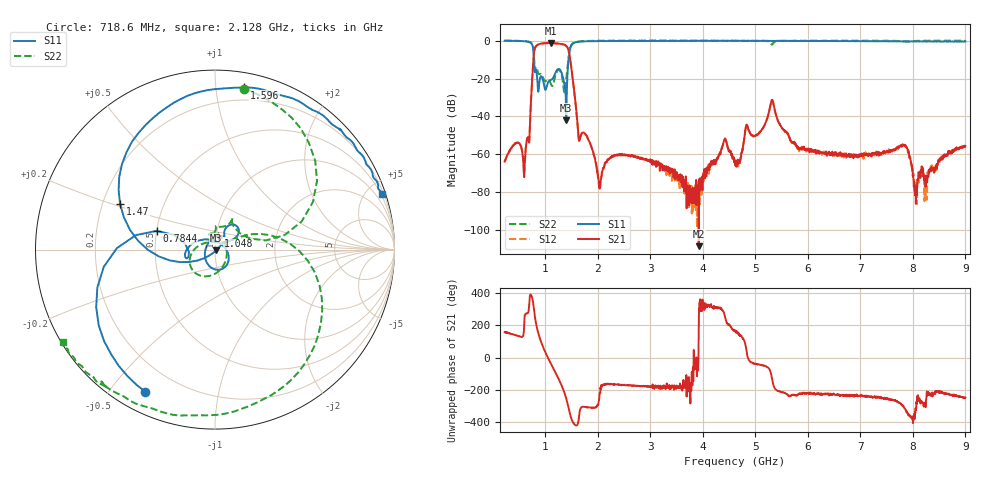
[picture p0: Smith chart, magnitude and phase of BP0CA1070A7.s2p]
!Agilent Technologies,E8358A,US41080443,A.07.50.56
!Agilent E8358A: A.07.50.56
!Date: Thursday, November 09, 2017 08:34:48
!Correction: S11(Full 2 Port(1,2))
!S21(Full 2 Port(1,2))
!S12(Full 2 Port(1,2))
!S22(Full 2 Port(1,2))
!S2P File: Measurements: S11, S21, S12, S22:
# Hz S  dB  R 50
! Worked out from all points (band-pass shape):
!   1601 points, 225 MHz to 9 GHz, reference 50 ohm
!   highest |S21| = -1.22 dB at 1.113 GHz (marker M1); lowest = -108.4 dB at 3.921 GHz (marker M2)
!   |S21| within 3 dB of the highest: 798.9 MHz to 1.432 GHz (632.8 MHz wide, 56.7 % of centre)
!   lowest |S11| = -42.0 dB at 1.399 GHz (marker M3), VSWR 1.02, Z = 50.7 - j0.309 ohm
!   |S11| at or under -10 dB: 785.7 MHz to 1.443 GHz (656.9 MHz wide, 59 % of centre)
!   |S22| runs from -27.3 to 0.1 dB; largest |S21 - S12| = 0.016
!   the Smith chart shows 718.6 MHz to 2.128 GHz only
!   S11 on the Smith chart (normalised r, x): 718.6 MHz: 0.09, -0.62; 784.4 MHz: 0.50, +0.12; 1.048 GHz: 1.02, +0.15; 1.47 GHz: 0.27, +0.21; 1.596 GHz: 0.10, +1.19; 2.128 GHz: 0.38, +6.17
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2.25e8  -0.07 -17.4  -63.77 157.8  -64.06 155.7  -0.01 163.2
5.979375e8  -0.32 -67.4  -72.06 -148.2  -70.46 -144.5  -0.25 119.2
7.185938e8  -1.09 -116.2  -36.68 31.4  -36.88 31.5  -0.81 79.6
7.844062e8  -9.32 162.2  -6.64 -59.8  -6.79 -59.5  -8.03 11.8
9.27e8  -18.85 -80.1  -1.54 91.4  -1.69 91.6  -17.93 87.7
1.047656e9  -22.38 77.6  -1.24 1.1  -1.39 1.3  -20.65 106.2
1.113469e9  -20.69 54.5  -1.22 -41.5  -1.38 -41.3  -23.26 49.8
1.294453e9  -15.94 34.7  -1.69 -160.3  -1.83 -160.1  -16.64 -161.5
1.398656e9  -41.95 -22.4  -2.73 107.0  -2.88 107.0  -20.44 30.4
1.469953e9  -4.64 154.4  -9.12 11.1  -9.26 10.9  -4.24 -18.6
1.596094e9  -0.74 79.7  -38.49 -59.8  -38.67 -60.0  -0.68 -92.7
1.689328e9  -0.46 58.4  -49.12 52.5  -49.34 53.9  -0.38 -114.2
2.128078e9  -0.17 18.4  -65.75 -168.1  -65.46 -168.9  -0.08 -148.7
3.153656e9  -0.16 -18.3  -65.06 -173.2  -65.67 178.0  0.09 -170.0
3.921469e9  -0.13 -32.8  -108.45 141.5  -74.74 -87.9  -0.01 -180.0
4.415062e9  -0.07 -38.4  -52.28 -95.3  -52.55 -95.8  -0.08 170.4
4.6125e9  -0.06 -40.5  -65.23 170.6  -62.72 172.2  -0.03 166.5
5.3145e9  -0.20 -47.0  -31.34 -124.0  -31.33 -123.8  -2.10 149.1
6.076828e9  -0.15 -55.8  -58.81 137.3  -58.21 139.3  -0.08 132.4
7.541156e9  -0.38 -87.0  -58.42 100.7  -57.28 103.3  -0.09 112.4
8.056688e9  -0.45 -103.3  -86.04 34.5  -76.94 -22.9  -0.19 111.8
9e9  -0.42 -132.4  -55.60 112.4  -55.62 109.3  -0.04 104.4
